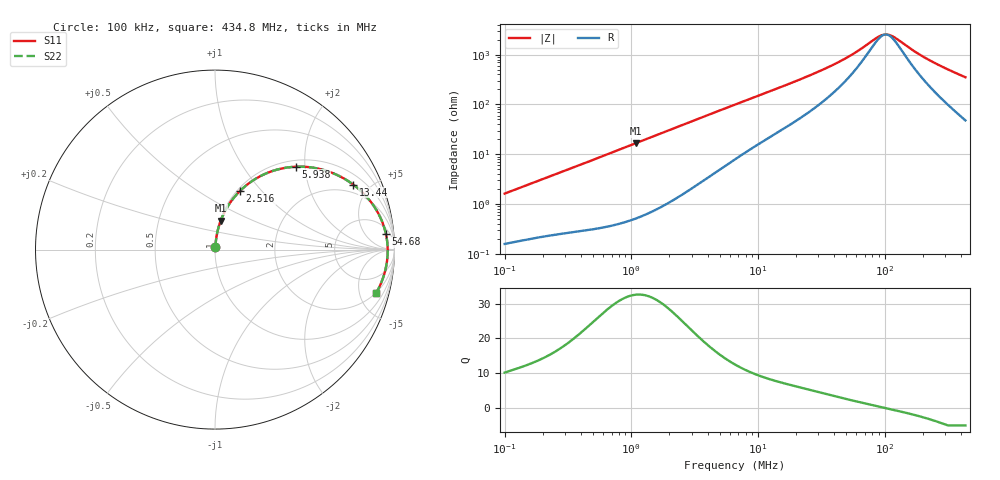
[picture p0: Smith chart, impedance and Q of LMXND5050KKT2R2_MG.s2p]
! LMXND5050KKT2R2_MG  S-PARAMETER MODEL  ( General Type )
! Model Generated by TAIYO YUDEN Corporation (http://www.ty-top.com)
! Version 1.0
! TAIYO YUDEN Control No. 191023NI43SB-FBB
! Copyright(c) 2019 TAIYO YUDEN CO.,LTD. All Rights Reserved.
! Product Description (link to TY-COMPAS)
! https://ds.yuden.co.jp/TYCOMPAS/or/detail?pn=LMXND5050KKT2R2NMG&u=M
! Products Name : Inductors
! Characteristics :
!  Inductance : 2.2 uH , SRF(min) : 65 MHz , DC Resistance(max) : 0.126 Ohm
!  Rated Current : Saturation :1500 mA , Temp Rise : 1400 mA
!  Case Size : 4.9 x 4.9 / 0.193 x 0.193 [mm/inch] , Thickness : 1 / 0.039 [mm/inch]
!  (Conditions: Temperature = 25 degC , DC Bias Current/Voltage = 0A / 0V)
! External Node Assignments :
!  1  o---GGG---o  2
! GND o---------o GND
! Frequency Range : 0.1MHz  -  434.768421MHz  [ 402 STEP ]
# MHz S RI R 50
! Freq[MHz].  S11 Real  S11 Imag  S21 Real  S21 Imag  S12 Real  S12 Imag  S22 Real  S22 Imag
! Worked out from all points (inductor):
!   401 points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, 100 kHz to 434.8 MHz, reference 50 ohm
!   read as one part in series: L = 2.55 uH near 104.3 kHz
!   highest Q = 32.6 at 1.089 MHz (marker M1), where L = 2.44 uH
!   self-resonance near 102.2 MHz
!   S11 on the Smith chart (normalised r, x): 100 kHz: 1.00, +0.03; 2.516 MHz: 1.03, +0.77; 5.938 MHz: 1.13, +1.79; 13.44 MHz: 1.50, +3.94; 54.68 MHz: 9, +18; 434.8 MHz: 1.96, -6.98
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0.1  0.00184 0.0161  0.9982 -0.0161  0.9982 -0.0161  0.00184 0.0161
0.406826  0.00679 0.0624  0.9932 -0.0624  0.9932 -0.0624  0.00679 0.0624
1.088688  0.0319 0.161  0.9681 -0.161  0.9681 -0.161  0.0319 0.161
1.65507  0.0673 0.2347  0.9327 -0.2347  0.9327 -0.2347  0.0673 0.2347
2.516108  0.1388 0.3264  0.8612 -0.3264  0.8612 -0.3264  0.1388 0.3264
3.745817  0.2569 0.4115  0.7431 -0.4115  0.7431 -0.4115  0.2569 0.4115
5.938145  0.45 0.4619  0.55 -0.4619  0.55 -0.4619  0.45 0.4619
6.733248  0.5068 0.461  0.4932 -0.461  0.4932 -0.461  0.5068 0.461
9.21848  0.6411 0.432  0.3589 -0.432  0.3589 -0.432  0.6411 0.432
13.43943  0.7704 0.3621  0.2296 -0.3621  0.2296 -0.3621  0.7704 0.3621
18.78933  0.8506 0.2875  0.1494 -0.2875  0.1494 -0.2875  0.8506 0.2875
26.82484  0.905 0.2105  0.095 -0.2105  0.095 -0.2105  0.905 0.2105
39.93507  0.9389 0.1353  0.0611 -0.1353  0.0611 -0.1353  0.9389 0.1353
54.67504  0.9528 0.085  0.0472 -0.085  0.0472 -0.085  0.9528 0.085
90.38256  0.9617 0.0159  0.0383 -0.0159  0.0383 -0.0159  0.9617 0.0159
100.3605  0.9622 0.00232  0.0378 -0.00232  0.0378 -0.00232  0.9622 0.00232
109.1303  0.9622 -0.00853  0.0378 0.00853  0.0378 0.00853  0.9622 -0.00853
121.178  0.9619 -0.0222  0.0381 0.0222  0.0381 0.0222  0.9619 -0.0222
169.4158  0.9578 -0.068  0.0422 0.068  0.0422 0.068  0.9578 -0.068
222.432  0.9501 -0.1099  0.0499 0.1099  0.0499 0.1099  0.9501 -0.1099
317.5582  0.9301 -0.1746  0.0699 0.1746  0.0699 0.1746  0.9301 -0.1746
434.7684  0.8971 -0.2429  0.1029 0.2429  0.1029 0.2429  0.8971 -0.2429
